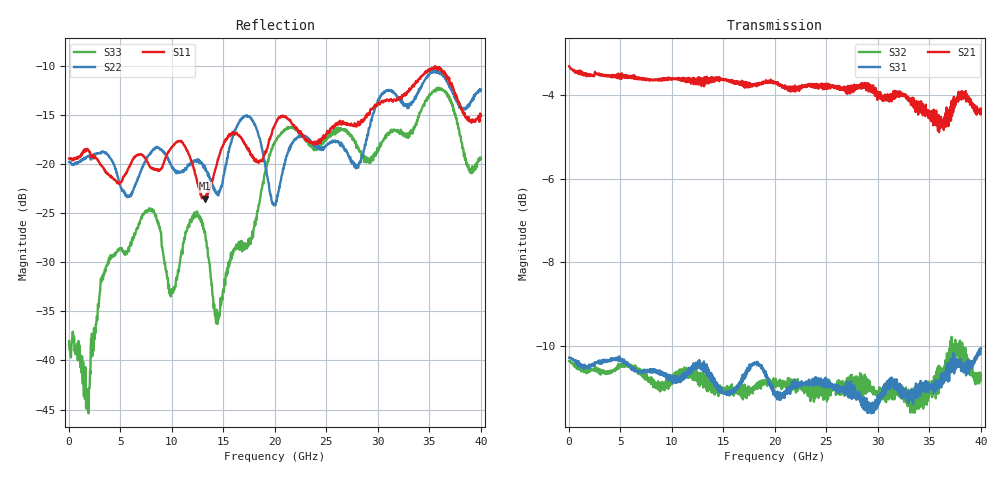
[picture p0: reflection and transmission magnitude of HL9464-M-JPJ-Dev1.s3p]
! 3/9/2020 11:23:47 AM
! H:\PRODUCTION_DATA\TEMP_S3P.S3P
! CHANNEL.1
! TR.MEASUREMENT
! CORRECTED.DATA
# GHZ S RI R 50.0
! FREQ.GHZ  S11RE  S11IM  S12RE  S12IM  S13RE  S13IM
!  S21RE  S21IM  S22RE  S22IM  S23RE  S23IM
!  S31RE  S31IM  S32RE  S32IM  S33RE  S33IM
!; PortSelection: Port_123
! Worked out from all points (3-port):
!   1143 points, 35 MHz to 40.01 GHz, reference 50 ohm
!   strongest paths, dB at 35 MHz, 10.01 GHz, 20.02 GHz, 30.03 GHz, 40.01 GHz:
!     S21: -3.3, -3.6, -3.7, -3.9, -4.3
!     S31: -10.3, -10.9, -11.1, -11.4, -10.1
!     S32: -10.4, -10.9, -10.8, -11.2, -10.8
!   lowest |S11| = -23.5 dB at 13.2 GHz (marker M1), VSWR 1.14, Z = 43.8 - j0.17 ohm
!   |S11| at or under -10 dB: start of sweep to end of sweep
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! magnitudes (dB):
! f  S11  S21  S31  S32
! 35 MHz  -19.5  -3.3  -10.3  -10.4
! 1.855 GHz  -18.6  -3.5  -10.5  -10.6
! 3.255 GHz  -20.3  -3.5  -10.3  -10.6
! 7.42 GHz  -19.4  -3.6  -10.6  -10.7
! 9.94 GHz  -18.4  -3.6  -10.7  -10.7
! 13.2 GHz  -23.5  -3.6  -10.6  -10.8
! 14.46 GHz  -19.6  -3.6  -11.0  -11.0
! 17.32 GHz  -18.3  -3.8  -10.5  -11.0
! 20.02 GHz  -16.0  -3.7  -11.1  -10.8
! 40.01 GHz  -15.1  -4.3  -10.1  -10.8
